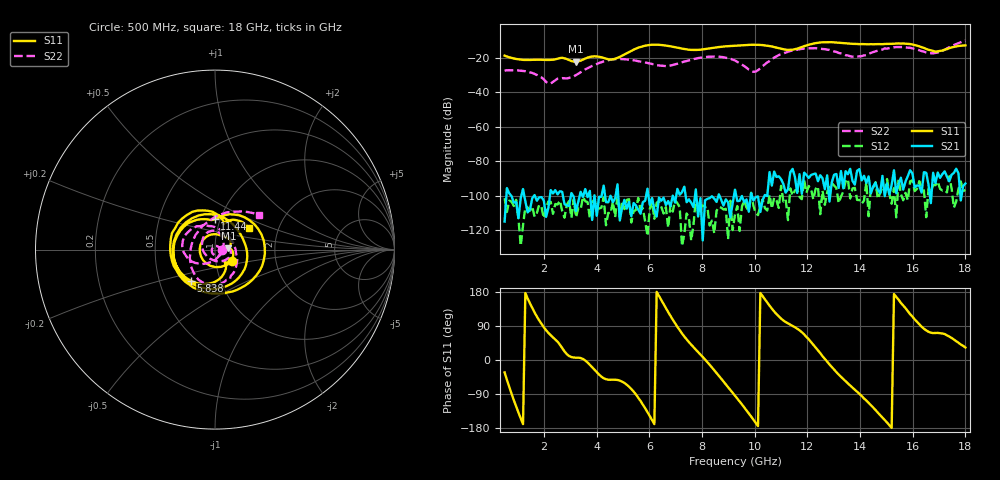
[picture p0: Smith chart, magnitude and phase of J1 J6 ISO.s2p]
!Agilent Technologies,N5230A,MY45001360,A.07.50.67
!Agilent N5230A: A.07.50.67
!Date: Tuesday, April 16, 2024 17:44:54
!Correction: S11(Full 2 Port(1,2))
!S21(Full 2 Port(1,2))
!S12(Full 2 Port(1,2))
!S22(Full 2 Port(1,2))
!S2P File: Measurements: S11, S21, S12, S22:
# Hz S  dB  R 50
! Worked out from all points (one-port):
!   201 points, 500 MHz to 18 GHz, reference 50 ohm
!   lowest |S11| = -22.4 dB at 3.212 GHz (marker M1), VSWR 1.16, Z = 58.1 + j0.937 ohm
!   |S11| at or under -10 dB: start of sweep to end of sweep
!   S11 on the Smith chart (normalised r, x): 500 MHz: 1.20, -0.15; 5.838 GHz: 0.72, -0.27; 11.44 GHz: 0.94, +0.33; 18 GHz: 1.41, +0.36
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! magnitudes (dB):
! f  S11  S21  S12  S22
! 500 MHz  -18.9  -114.9  -101.4  -27.6
! 1.55 GHz  -21.3  -101.4  -106.3  -28.9
! 2.163 GHz  -21.4  -107.0  -103.3  -35.0
! 2.688 GHz  -20.1  -97.8  -108.8  -31.9
! 3.212 GHz  -22.4  -109.0  -112.4  -30.1
! 3.475 GHz  -21.2  -100.8  -100.7  -27.8
! 3.913 GHz  -19.3  -99.7  -102.3  -24.3
! 4.612 GHz  -21.1  -103.8  -103.4  -21.0
! 5.838 GHz  -13.1  -102.9  -114.8  -22.8
! 6.362 GHz  -12.6  -101.1  -103.2  -24.6
! 7.5 GHz  -15.5  -102.1  -112.8  -21.6
! 8.2 GHz  -14.9  -101.8  -106.6  -19.6
! 9.25 GHz  -13.1  -96.5  -110.9  -21.7
! 10.04 GHz  -12.6  -100.8  -110.3  -28.1
! 10.74 GHz  -14.0  -86.0  -101.1  -20.0
! 11.44 GHz  -15.4  -84.5  -99.9  -15.9
! 12.22 GHz  -12.0  -87.5  -102.1  -14.6
! 13.8 GHz  -12.1  -93.6  -95.4  -19.5
! 15.11 GHz  -12.1  -99.4  -99.0  -14.6
! 15.9 GHz  -12.2  -85.2  -91.7  -14.4
! 16.77 GHz  -16.2  -86.7  -93.8  -17.5
! 18 GHz  -12.9  -93.0  -96.6  -10.1
